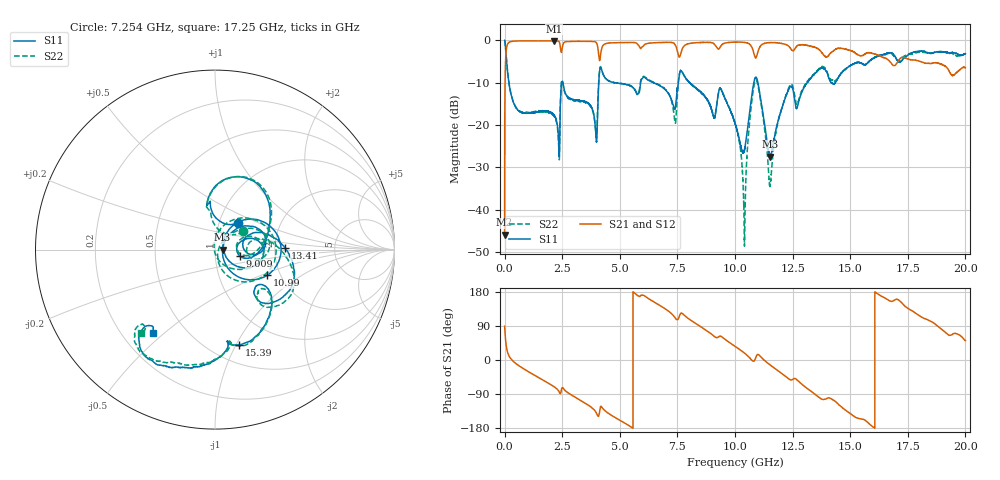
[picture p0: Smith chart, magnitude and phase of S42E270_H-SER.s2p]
!{S42E270}
!Johanson Technology Inc.
!www.johansontechnology.com
!Test Board Conditions:
!Substrate Type  RO4350B
!Substrate Thickness  50 mil
!Substrate Dk  3.66
!TL Type: GCPW
!TL Trace Width  60 mil
!TL Gap  10 mil
!Electrode orientation  Horizontal
!DUT TOPOLOGY	SERIES
!Mounting Pad LxW  14x55 mil
! Created Wed Nov 25 22:08:28 2020
# khz S ma R 50
! 2 Port Network Data from SP1.SP block
! freq  magS11  angS11  magS21  angS21  magS12  angS12  magS22  angS22
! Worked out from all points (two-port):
!   20001 points, 300 kHz to 20 GHz, reference 50 ohm
!   highest |S21| = -0.10 dB at 2.14 GHz (marker M1); lowest = -46.0 dB at 300 kHz (marker M2)
!   |S21| within 3 dB of the highest: 58.65 MHz to 4.079 GHz (4.02 GHz wide, 194 % of centre); 4.174 GHz to 7.525 GHz (3.351 GHz wide, 57.3 % of centre)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
!   lowest |S11| = -27.5 dB at 11.53 GHz (marker M3), VSWR 1.09, Z = 54.4 - j0.118 ohm
!   |S11| at or under -10 dB: 186.3 MHz to 2.467 GHz (2.281 GHz wide, 172 % of centre); 8.037 GHz to 10.82 GHz (2.779 GHz wide, 29.5 % of centre); 10.99 GHz to 13.13 GHz (2.133 GHz wide, 17.7 % of centre)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
!   |S22| runs from -48.7 to 0.0 dB; largest |S21 - S12| = 0.017
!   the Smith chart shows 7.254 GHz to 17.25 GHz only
!   S11 on the Smith chart (normalised r, x): 7.254 GHz: 1.22, +0.38; 9.009 GHz: 1.32, -0.10; 10.99 GHz: 1.71, -0.55; 13.41 GHz: 2.28, +0.05; 15.39 GHz: 0.68, -1.03; 17.25 GHz: 0.33, -0.46
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300  0.9997 -0.5  0.00504 88.9  0.005102 89.7  0.9969 -0.2
102300  0.5059 -63.4  0.8603 26.6  0.8608 26.5  0.5078 -63.3
164300  0.35 -75.7  0.9349 14.3  0.9347 14.3  0.3524 -75.6
2140300  0.1316 -159.9  0.9891 -70.3  0.9881 -70.3  0.1271 -159.5
3334300  0.1935 158.3  0.9768 -107.9  0.9763 -107.9  0.1889 165.9
5194300  0.3045 103.6  0.9441 -165.9  0.9439 -165.9  0.3057 105.7
6667300  0.298 59.9  0.9424 146.4  0.941 146.4  0.302 56.3
7254300  0.1949 49.9  0.9446 121.7  0.9444 121.7  0.189 33.4
7685300  0.431 53.8  0.7611 123.8  0.7586 123.9  0.4344 51.3
9009300  0.1422 -14.5  0.9377 67.0  0.9396 66.9  0.1437 -9.9
1.00003e7  0.1048 -39.2  0.9547 36.1  0.9571 36.2  0.1071 -57.8
1.04093e7  0.05074 24.8  0.9475 18.3  0.9467 18.3  0.004195 -157.2
1.07363e7  0.2286 45.9  0.8281 -0.9  0.8263 -0.7  0.1978 57.8
1.09853e7  0.3238 -26.3  0.7182 14.7  0.7207 14.9  0.3032 -30.0
1.15313e7  0.04201 -1.5  0.9434 -13.4  0.9427 -13.3  0.01972 -1.3
1.23123e7  0.2575 29.1  0.8646 -48.8  0.8667 -48.7  0.2664 23.8
1.33343e7  0.3695 5.3  0.8465 -83.8  0.8505 -83.7  0.3763 -2.1
1.34073e7  0.3902 1.3  0.8404 -87.3  0.8411 -87.0  0.3947 -5.2
1.53933e7  0.5464 -75.7  0.6653 -154.7  0.6667 -155.1  0.5551 -74.9
1.66673e7  0.7094 -114.5  0.5853 157.6  0.5712 157.7  0.7042 -120.3
1.72503e7  0.5803 -126.8  0.6306 149.7  0.6227 149.5  0.6219 -131.3
2e7  0.6994 145.2  0.474 50.8  0.4778 51.6  0.6846 136.5
